(* Logix 5000 AddOnInstructionDefinition export B256_MODINV; software revision 30.00 *)

ADD_ON_INSTRUCTION D_SHR   (* revision 1.0, vendor Ken Fischer, NSWCPD, C512 *)
// DINT bit shift right of the 32-bit argument Inp_A by Inp_B bits with paddding by zeros on the right
// Revision note:
// Rev1.0: TBD - Initial Release
VAR_IN_OUT
   Inp_A : DINT; {required}   // 64-bit Integer to be right circular rotated
END_VAR
VAR_INPUT
   Inp_B : INT; {required}   // Number of bits to shift
END_VAR
VAR_IN_OUT
   Out : DINT; {required}   // Result
END_VAR
VAR
   BSR_Cntrl : CONTROL := (LEN := 32);
   ONS : BOOL;
   Source_Bit : BOOL;
   Wrk_InpA : DINT[2];
END_VAR

ROUTINE Logic   (* ladder *)
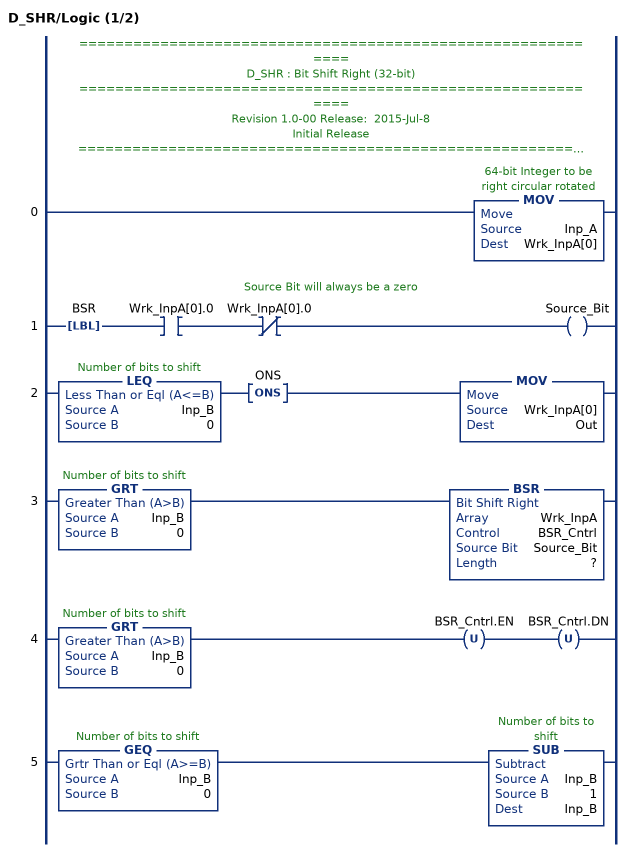
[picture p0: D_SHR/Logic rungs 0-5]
   // ============================================================
   // D_SHR : Bit Shift Right (32-bit)
   // ============================================================
   // Revision 1.0-00 Release:  2015-Jul-8
   // Initial Release
   // ============================================================
   // Performs a right bit shift of the 32-bit argument Inp_A by the
   // number of bits defined in the 16-bit argument Inp_B, with padding by zeros.
   0: MOV(Inp_A,Wrk_InpA[0]);
   // Source Bit will always be a zero
   1: LBL(BSR)XIC(Wrk_InpA[0].0)XIO(Wrk_InpA[0].0)OTE(Source_Bit);
   2: LEQ(Inp_B,0)ONS(ONS)MOV(Wrk_InpA[0],Out);
   3: GRT(Inp_B,0)BSR(Wrk_InpA,BSR_Cntrl,Source_Bit,?);
   4: GRT(Inp_B,0)OTU(BSR_Cntrl.EN)OTU(BSR_Cntrl.DN);
   5: GEQ(Inp_B,0)SUB(Inp_B,1,Inp_B);
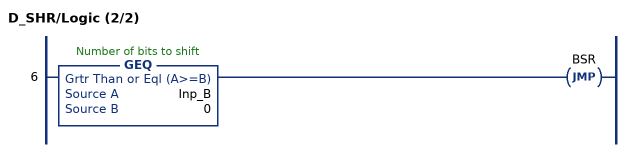
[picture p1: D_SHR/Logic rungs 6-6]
   6: GEQ(Inp_B,0)JMP(BSR);
END_ROUTINE
END_ADD_ON_INSTRUCTION

ADD_ON_INSTRUCTION B256_NRED   (* revision 1.0 20170916, vendor Kenneth A. Fischer *)
// Reduce 256-bit integer stored in 22 pieces by propagating carries
// Revision note:
// Rev1.0: 20170916 - Initial Release
VAR_IN_OUT
   Inp_C : DINT[22]; {required}
END_VAR
VAR
   D_SHR : D_SHR;
   temp : DINT;
   i : INT;
END_VAR

ROUTINE Logic   (* ladder *)
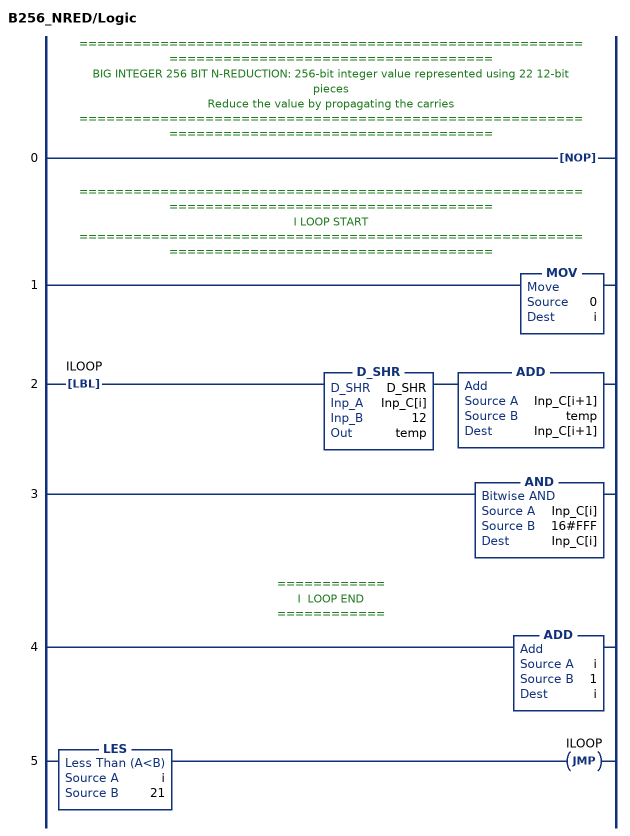
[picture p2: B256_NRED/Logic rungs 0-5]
   // ============================================================================================
   // BIG INTEGER 256 BIT N-REDUCTION: 256-bit integer value represented using 22 12-bit pieces
   // Reduce the value by propagating the carries
   // ============================================================================================
   0: NOP();
   // ============================================================================================
   // I LOOP START
   // ============================================================================================
   1: MOV(0,i);
   2: LBL(ILOOP)D_SHR(D_SHR,Inp_C[i],12,temp)ADD(Inp_C[i+1],temp,Inp_C[i+1]);
   3: AND(Inp_C[i],16#FFF,Inp_C[i]);
   // ============
   // I  LOOP END
   // ============
   4: ADD(i,1,i);
   5: LES(i,21)JMP(ILOOP);
END_ROUTINE
END_ADD_ON_INSTRUCTION

ADD_ON_INSTRUCTION B256_FRED   (* revision 1.0 20170916, vendor Kenneth A. Fischer *)
// fast_reduce:  reduce by propagating the carries starting at a particular offset and stoping once the carry becomes zero
// Revision note:
// Rev1.0: 20170916 - Initial Release
VAR_IN_OUT
   Inp_C : DINT[22]; {required}
END_VAR
VAR_INPUT
   Inp_offset : INT; {required}
END_VAR
VAR
   i : INT;
   carry : DINT;
   D_SHR : D_SHR;
END_VAR

ROUTINE Logic   (* ladder *)
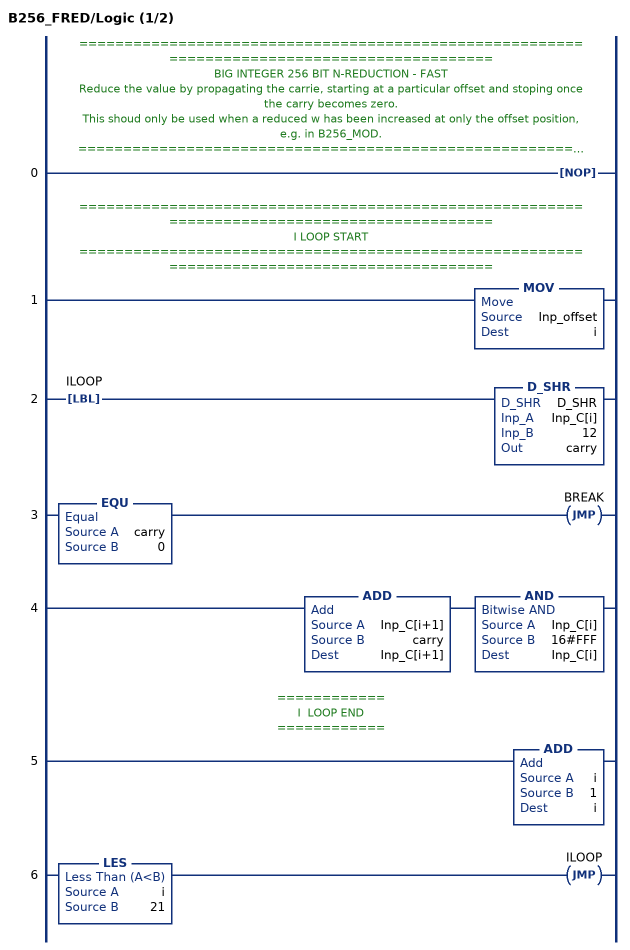
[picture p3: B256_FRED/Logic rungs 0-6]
   // ============================================================================================
   // BIG INTEGER 256 BIT N-REDUCTION - FAST
   // Reduce the value by propagating the carrie, starting at a particular offset and stoping once the carry becomes zero.
   // This shoud only be used when a reduced w has been increased at only the offset position, e.g. in B256_MOD.
   // ============================================================================================
   0: NOP();
   // ============================================================================================
   // I LOOP START
   // ============================================================================================
   1: MOV(Inp_offset,i);
   2: LBL(ILOOP)D_SHR(D_SHR,Inp_C[i],12,carry);
   3: EQU(carry,0)JMP(BREAK);
   4: ADD(Inp_C[i+1],carry,Inp_C[i+1])AND(Inp_C[i],16#FFF,Inp_C[i]);
   // ============
   // I  LOOP END
   // ============
   5: ADD(i,1,i);
   6: LES(i,21)JMP(ILOOP);
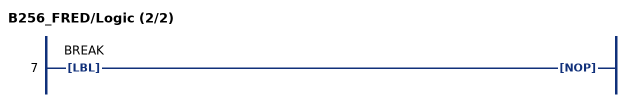
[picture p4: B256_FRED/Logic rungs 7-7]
   7: LBL(BREAK)NOP();
END_ROUTINE
END_ADD_ON_INSTRUCTION

ADD_ON_INSTRUCTION D_SHL   (* revision 1.0, vendor Ken Fischer, NSWCPD, C512 *)
// DINT bit shift left of the 32-bit argument Inp_A by Inp_B bits with paddding by zeros on the right
// Revision note:
// Rev1.0: TBD - Initial Release
VAR_IN_OUT
   Inp_A : DINT; {required}   // 64-bit Integer to be right circular rotated
END_VAR
VAR_INPUT
   Inp_B : INT; {required}   // Number of bits to shift
END_VAR
VAR_IN_OUT
   Out : DINT; {required}   // Result
END_VAR
VAR
   Wrk_InpA : DINT[2];
   Source_Bit : BOOL;
   ONS : BOOL;
   BSL_Cntrl : CONTROL := (LEN := 32);
END_VAR

ROUTINE Logic   (* ladder *)
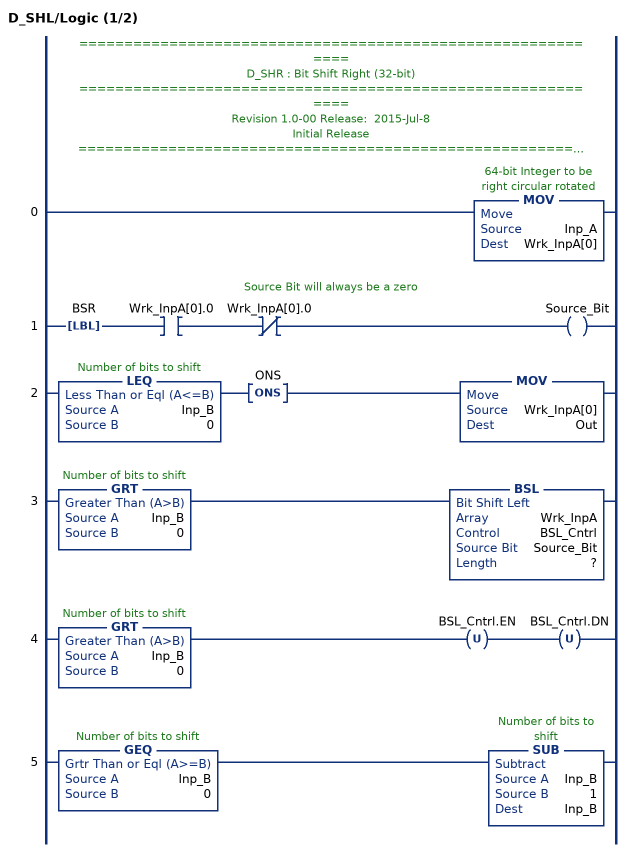
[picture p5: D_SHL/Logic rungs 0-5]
   // ============================================================
   // D_SHR : Bit Shift Right (32-bit)
   // ============================================================
   // Revision 1.0-00 Release:  2015-Jul-8
   // Initial Release
   // ============================================================
   // Performs a left bit shift of the 32-bit argument Inp_A by the
   // number of bits defined in the 16-bit argument Inp_B, with padding by zeros.
   0: MOV(Inp_A,Wrk_InpA[0]);
   // Source Bit will always be a zero
   1: LBL(BSR)XIC(Wrk_InpA[0].0)XIO(Wrk_InpA[0].0)OTE(Source_Bit);
   2: LEQ(Inp_B,0)ONS(ONS)MOV(Wrk_InpA[0],Out);
   3: GRT(Inp_B,0)BSL(Wrk_InpA,BSL_Cntrl,Source_Bit,?);
   4: GRT(Inp_B,0)OTU(BSL_Cntrl.EN)OTU(BSL_Cntrl.DN);
   5: GEQ(Inp_B,0)SUB(Inp_B,1,Inp_B);
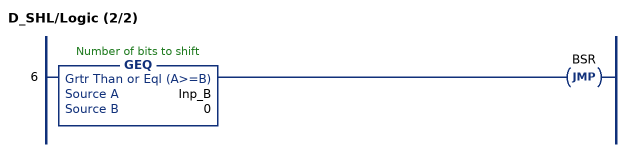
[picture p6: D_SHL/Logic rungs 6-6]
   6: GEQ(Inp_B,0)JMP(BSR);
END_ROUTINE
END_ADD_ON_INSTRUCTION

ADD_ON_INSTRUCTION B256_MOD   (* revision 1.0 20170916, vendor Kenneth A. Fischer *)
// c = d mod (2^255 - 19)
// Revision note:
// Rev1.0: 20170916 - Initial Release
VAR_IN_OUT
   Inp_D : DINT[43]; {required}
   Out_C : DINT[22]; {required}
END_VAR
VAR
   B256_NRED : B256_NRED;
   D_SHL : D_SHL;
   D_SHR : D_SHR;
   i : INT;
   t : DINT;
   temp : DINT;
   temp2 : DINT;
   B256_FRED : B256_FRED;
   offset : DINT;
END_VAR

ROUTINE Logic   (* ladder *)
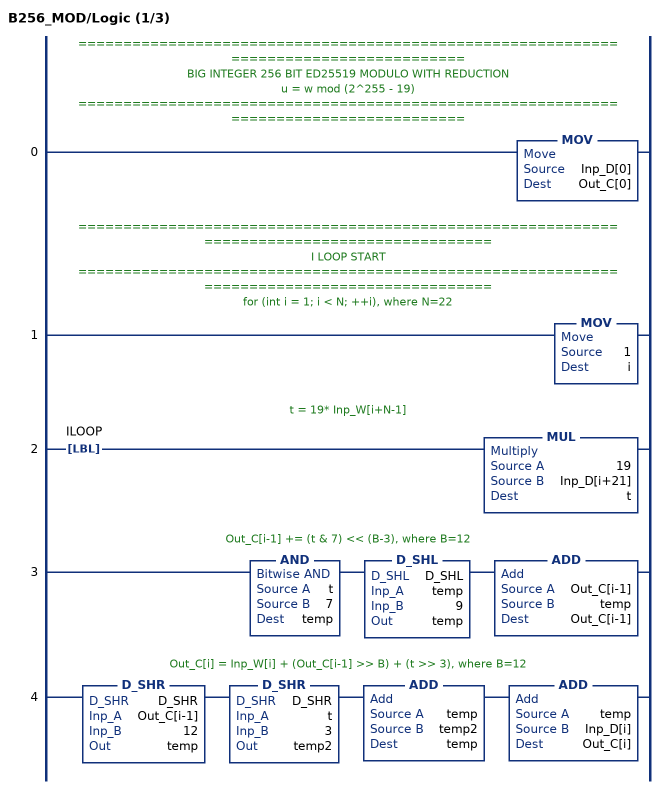
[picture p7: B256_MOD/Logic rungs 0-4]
   // ======================================================================================
   // BIG INTEGER 256 BIT ED25519 MODULO WITH REDUCTION
   //  u = w mod (2^255 - 19)
   // ======================================================================================
   0: MOV(Inp_D[0],Out_C[0]);
   // ============================================================================================
   // I LOOP START
   // ============================================================================================
   // for (int i = 1; i < N; ++i), where N=22
   1: MOV(1,i);
   // t = 19* Inp_W[i+N-1]
   2: LBL(ILOOP)MUL(19,Inp_D[i+21],t);
   // Out_C[i-1] += (t & 7) << (B-3), where B=12
   3: AND(t,7,temp)D_SHL(D_SHL,temp,9,temp)ADD(Out_C[i-1],temp,Out_C[i-1]);
   // Out_C[i] = Inp_W[i] + (Out_C[i-1] >> B) + (t >> 3), where B=12
   4: D_SHR(D_SHR,Out_C[i-1],12,temp)D_SHR(D_SHR,t,3,temp2)ADD(temp,temp2,temp)ADD(temp,Inp_D[i],Out_C[i]);
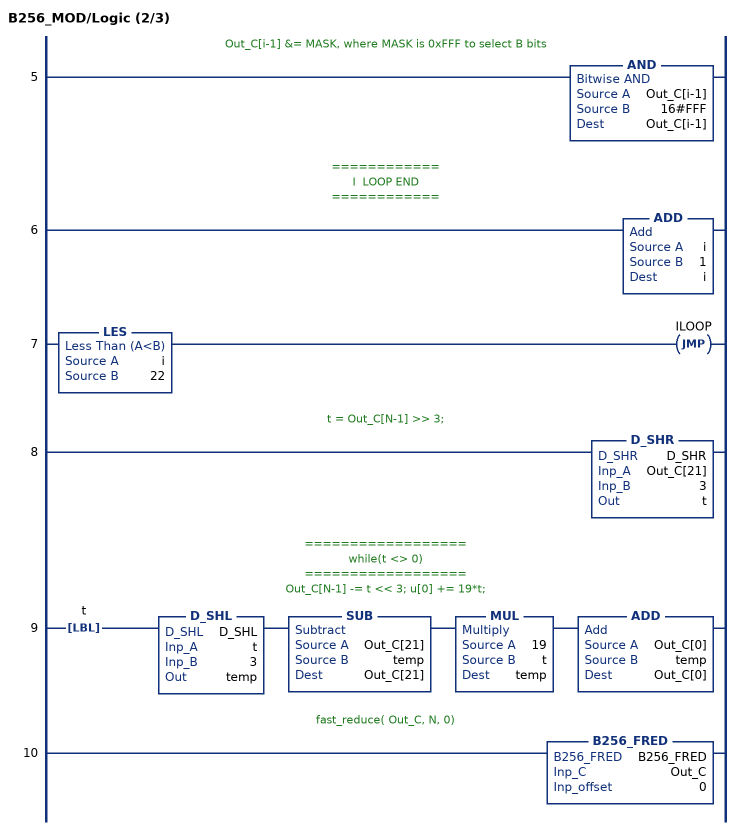
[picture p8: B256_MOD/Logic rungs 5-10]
   // Out_C[i-1] &= MASK, where MASK is 0xFFF to select B bits
   5: AND(Out_C[i-1],16#FFF,Out_C[i-1]);
   // ============
   // I  LOOP END
   // ============
   6: ADD(i,1,i);
   7: LES(i,22)JMP(ILOOP);
   // t = Out_C[N-1] >> 3;
   8: D_SHR(D_SHR,Out_C[21],3,t);
   // ==================
   // while(t <> 0)
   // ==================
   // Out_C[N-1] -= t << 3; u[0] += 19*t;
   9: LBL(t)D_SHL(D_SHL,t,3,temp)SUB(Out_C[21],temp,Out_C[21])MUL(19,t,temp)ADD(Out_C[0],temp,Out_C[0]);
   // fast_reduce( Out_C, N, 0)
   10: B256_FRED(B256_FRED,Out_C,0);
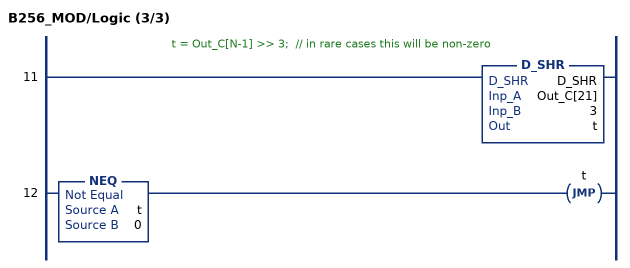
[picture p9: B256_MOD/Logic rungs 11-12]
   // t = Out_C[N-1] >> 3;  // in rare cases this will be non-zero
   11: D_SHR(D_SHR,Out_C[21],3,t);
   12: NEQ(t,0)JMP(t);
END_ROUTINE
END_ADD_ON_INSTRUCTION

ADD_ON_INSTRUCTION B256_NNRED   (* revision 1.0 20170916, vendor Kenneth A. Fischer *)
// Reduce 256-bit integer stored in 43 pieces by propagating carries
// Revision note:
// Rev1.0: 20170916 - Initial Release
VAR_IN_OUT
   Inp_D : DINT[43]; {required}
END_VAR
VAR
   temp : DINT;
   i : INT;
   D_SHR : D_SHR;
END_VAR

ROUTINE Logic   (* ladder *)
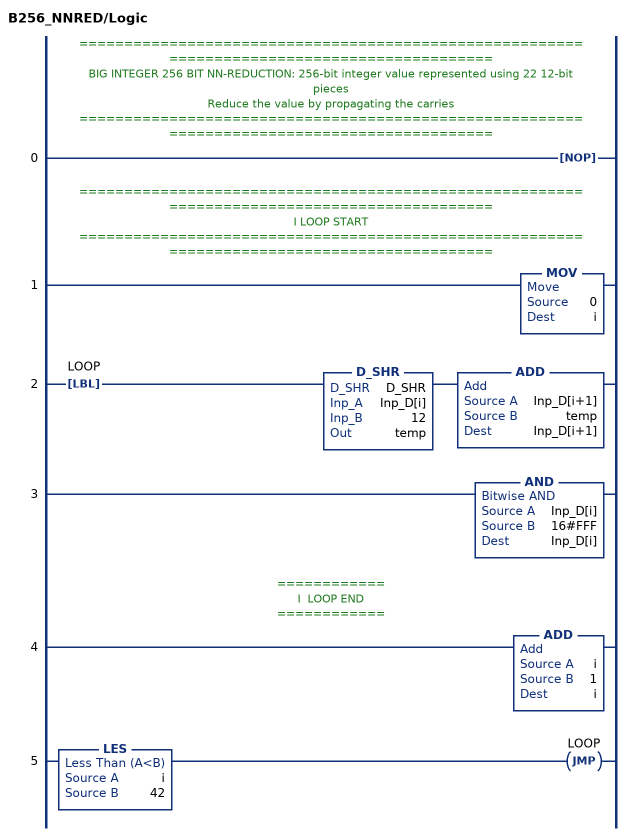
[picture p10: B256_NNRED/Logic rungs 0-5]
   // ============================================================================================
   // BIG INTEGER 256 BIT NN-REDUCTION: 256-bit integer value represented using 22 12-bit pieces
   // Reduce the value by propagating the carries
   // ============================================================================================
   0: NOP();
   // ============================================================================================
   // I LOOP START
   // ============================================================================================
   1: MOV(0,i);
   2: LBL(LOOP)D_SHR(D_SHR,Inp_D[i],12,temp)ADD(Inp_D[i+1],temp,Inp_D[i+1]);
   3: AND(Inp_D[i],16#FFF,Inp_D[i]);
   // ============
   // I  LOOP END
   // ============
   4: ADD(i,1,i);
   5: LES(i,42)JMP(LOOP);
END_ROUTINE
END_ADD_ON_INSTRUCTION

ADD_ON_INSTRUCTION B256_MUL   (* revision 1.0 20170916, vendor Kenneth A. Fischer *)
// c3 = c1*c2 with reduction and mod
// Revision note:
// Rev1.0: 20170916 - Initial Release
VAR_IN_OUT
   Temp_D : DINT[43]; {required}
   Inp_C1 : DINT[22]; {required}
   Inp_C2 : DINT[22]; {required}
   Out_C3 : DINT[22]; {required}
END_VAR
VAR
   B256_MOD : B256_MOD;
   B256_NNRED : B256_NNRED;
   i : INT;
   j : INT;
   mul_temp : DINT;
END_VAR

ROUTINE Logic   (* ladder *)
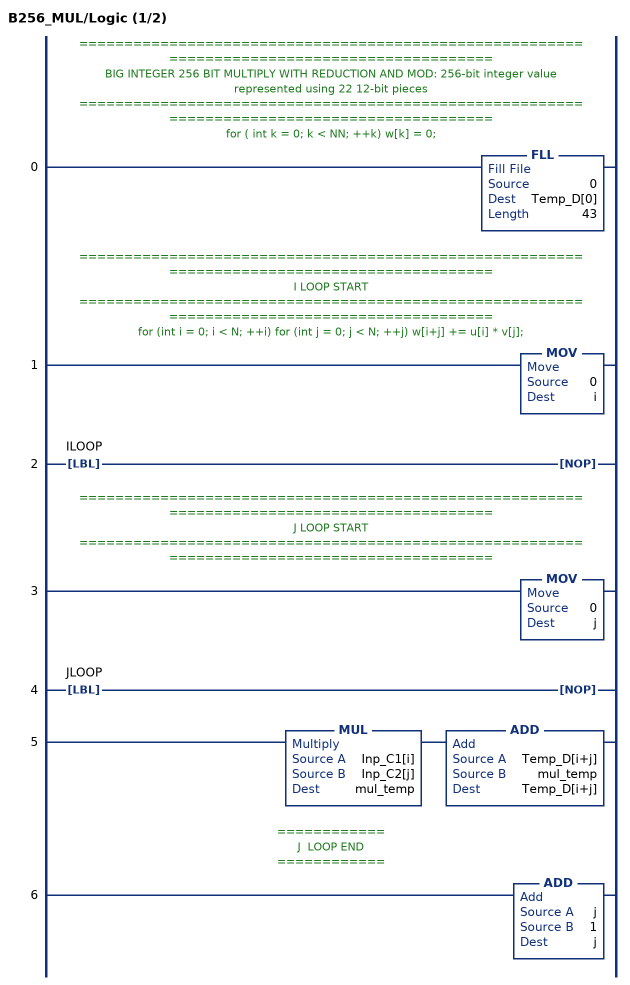
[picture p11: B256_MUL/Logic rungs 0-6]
   // ============================================================================================
   // BIG INTEGER 256 BIT MULTIPLY WITH REDUCTION AND MOD: 256-bit integer value represented using 22 12-bit pieces
   // ============================================================================================
   // for ( int k = 0; k < NN; ++k) w[k] = 0;
   0: FLL(0,Temp_D[0],43);
   // ============================================================================================
   // I LOOP START
   // ============================================================================================
   // for (int i = 0; i < N; ++i) for (int j = 0; j < N; ++j) w[i+j] += u[i] * v[j];
   1: MOV(0,i);
   2: LBL(ILOOP)NOP();
   // ============================================================================================
   // J LOOP START
   // ============================================================================================
   3: MOV(0,j);
   4: LBL(JLOOP)NOP();
   5: MUL(Inp_C1[i],Inp_C2[j],mul_temp)ADD(Temp_D[i+j],mul_temp,Temp_D[i+j]);
   // ============
   // J  LOOP END
   // ============
   6: ADD(j,1,j);
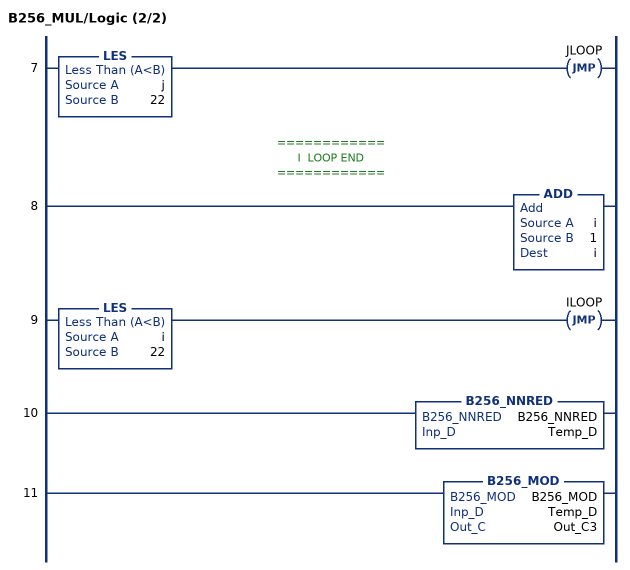
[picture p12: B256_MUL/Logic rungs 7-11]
   7: LES(j,22)JMP(JLOOP);
   // ============
   // I  LOOP END
   // ============
   8: ADD(i,1,i);
   9: LES(i,22)JMP(ILOOP);
   10: B256_NNRED(B256_NNRED,Temp_D);
   11: B256_MOD(B256_MOD,Temp_D,Out_C3);
END_ROUTINE
END_ADD_ON_INSTRUCTION

ADD_ON_INSTRUCTION B256_SQU   (* revision 1.0 20170916, vendor Kenneth A. Fischer *)
// c2 = c1*c1 with reduction and mod
// uses about half the number of multiplies compared to B256_MOD
// Revision note:
// Rev1.0: 20170916 - Initial Release
VAR_IN_OUT
   Temp_D : DINT[43]; {required}
   Inp_C1 : DINT[22]; {required}
   Out_C2 : DINT[22]; {required}
END_VAR
VAR
   B256_NNRED : B256_NNRED;
   i : INT;
   j : INT;
   z : INT;
   mul_temp : DINT;
   B256_MOD : B256_MOD;
   B256_NRED : B256_NRED;
   t : DINT;
END_VAR

ROUTINE Logic   (* ladder *)
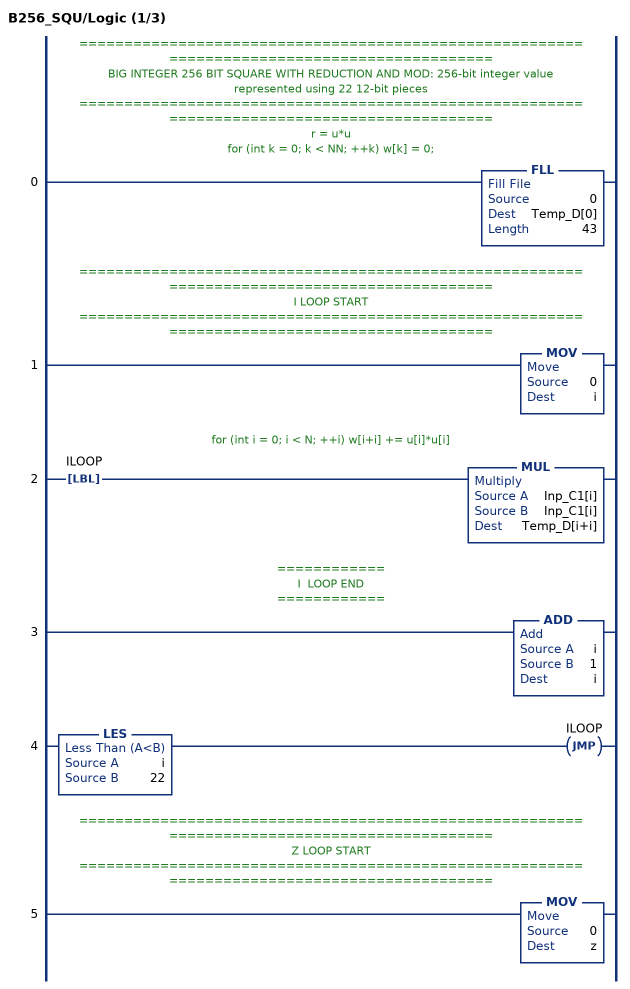
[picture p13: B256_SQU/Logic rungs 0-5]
   // ============================================================================================
   // BIG INTEGER 256 BIT SQUARE WITH REDUCTION AND MOD: 256-bit integer value represented using 22 12-bit pieces
   // ============================================================================================
   // r = u*u
   // for (int k = 0; k < NN; ++k) w[k] = 0;
   0: FLL(0,Temp_D[0],43);
   // ============================================================================================
   // I LOOP START
   // ============================================================================================
   1: MOV(0,i);
   // for (int i = 0; i < N; ++i) w[i+i] += u[i]*u[i]
   2: LBL(ILOOP)MUL(Inp_C1[i],Inp_C1[i],Temp_D[i+i]);
   // ============
   // I  LOOP END
   // ============
   3: ADD(i,1,i);
   4: LES(i,22)JMP(ILOOP);
   // ============================================================================================
   // Z LOOP START
   // ============================================================================================
   5: MOV(0,z);
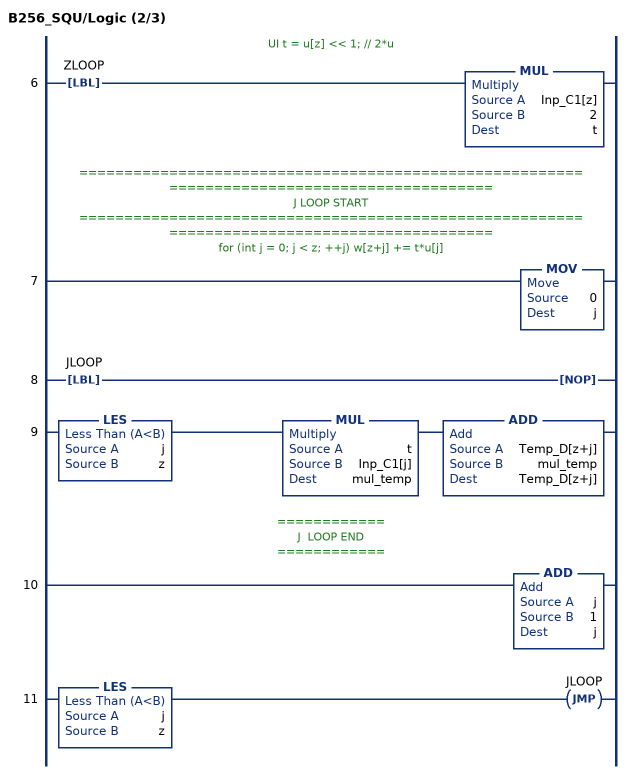
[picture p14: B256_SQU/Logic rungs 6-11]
   // UI t = u[z] << 1; // 2*u
   6: LBL(ZLOOP)MUL(Inp_C1[z],2,t);
   // ============================================================================================
   // J LOOP START
   // ============================================================================================
   // for (int j = 0; j < z; ++j) w[z+j] += t*u[j]
   7: MOV(0,j);
   8: LBL(JLOOP)NOP();
   9: LES(j,z)MUL(t,Inp_C1[j],mul_temp)ADD(Temp_D[z+j],mul_temp,Temp_D[z+j]);
   // ============
   // J  LOOP END
   // ============
   10: ADD(j,1,j);
   11: LES(j,z)JMP(JLOOP);
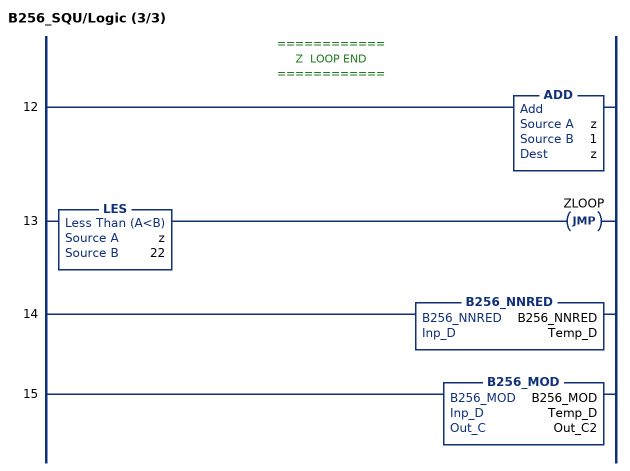
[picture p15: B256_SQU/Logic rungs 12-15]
   // ============
   // Z  LOOP END
   // ============
   12: ADD(z,1,z);
   13: LES(z,22)JMP(ZLOOP);
   14: B256_NNRED(B256_NNRED,Temp_D);
   15: B256_MOD(B256_MOD,Temp_D,Out_C2);
END_ROUTINE
END_ADD_ON_INSTRUCTION

ADD_ON_INSTRUCTION B256_MODINV   (* revision 1.0 20170916, vendor Kenneth A. Fischer *)
// c2 = c1^(m-2) mod m, m=2^255-19
// Revision note:
// Rev1.0: 20170916 - Initial Release
VAR_IN_OUT
   Temp_C1 : DINT[22]; {required}
   Temp_C2 : DINT[22]; {required}
   Temp_D : DINT[43]; {required}
   Temp_E : DINT[32]; {required}
   Inp_C1 : DINT[22]; {required}   // V
   Out_C2 : DINT[22]; {required}   // U
END_VAR
VAR_OUTPUT
   i : INT; {access Read Only}
END_VAR
VAR_INPUT
   SEQCTRL_RESET : BOOL;   // Resets Point Multiplication if Toggled True
END_VAR
VAR_OUTPUT
   SEQCTRL_DN : BOOL; {access Read Only}   // Complete
   SEQCTRL_STEP : INT; {access Read Only}
END_VAR
VAR
   SEQCTRL_CMD : INT;
   SEQCTRL_DONE : INT;
   SEQCTRL_CMD_TABLE : INT[35];
   SEQCTRL_NEXT_STEP : INT;
   TEMP : INT;
   j : INT;
   b : DINT;
   B256_MUL : B256_MUL;
   B256_SQU : B256_SQU;
END_VAR

ROUTINE Logic   (* ladder *)
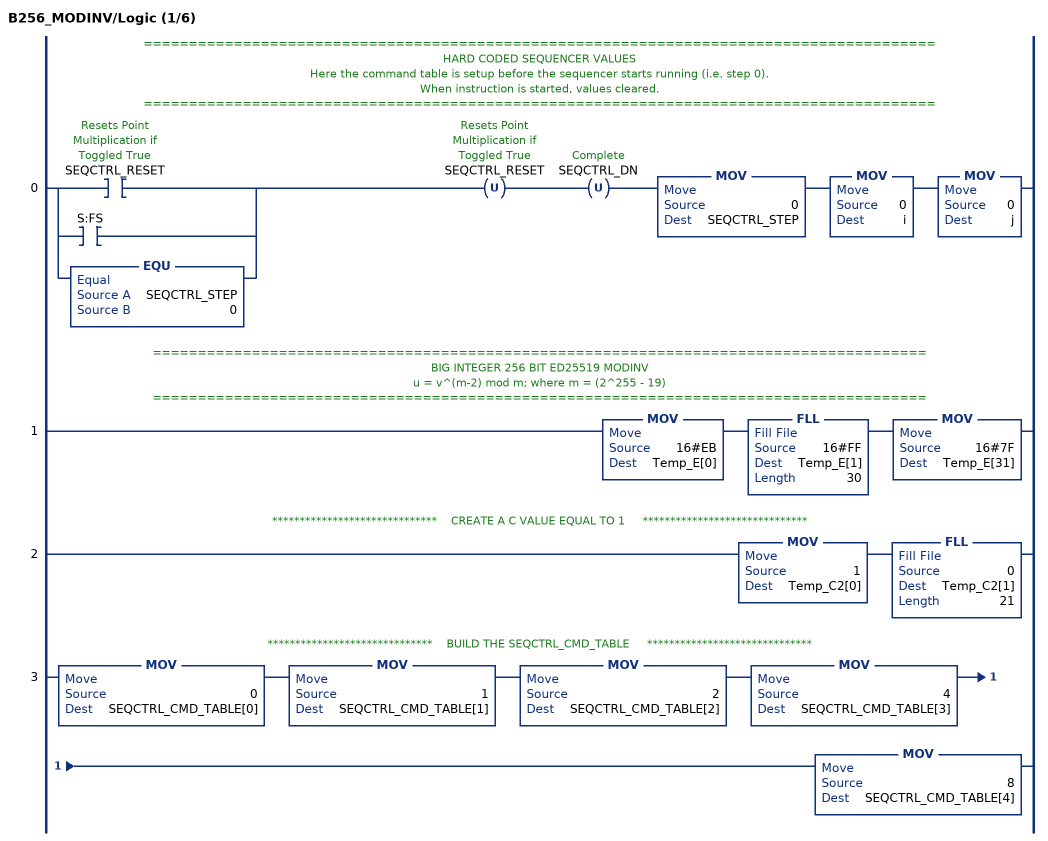
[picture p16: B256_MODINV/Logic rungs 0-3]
   // ========================================================================================
   // HARD CODED SEQUENCER VALUES
   // Here the command table is setup before the sequencer starts running (i.e. step 0).
   // When instruction is started, values cleared.
   // ========================================================================================
   0: [[XIC(SEQCTRL_RESET) ,XIC(S:FS) ] ,EQU(SEQCTRL_STEP,0) ]OTU(SEQCTRL_RESET)OTU(SEQCTRL_DN)MOV(0,SEQCTRL_STEP)MOV(0,i)MOV(0,j);
   // ======================================================================================
   // BIG INTEGER 256 BIT ED25519 MODINV
   //  u = v^(m-2) mod m; where m = (2^255 - 19)
   // ======================================================================================
   1: MOV(16#EB,Temp_E[0])FLL(16#FF,Temp_E[1],30)MOV(16#7F,Temp_E[31]);
   // ******************************    CREATE A C VALUE EQUAL TO 1     ******************************
   2: MOV(1,Temp_C2[0])FLL(0,Temp_C2[1],21);
   // ******************************    BUILD THE SEQCTRL_CMD_TABLE     ******************************
   3: MOV(0,SEQCTRL_CMD_TABLE[0])MOV(1,SEQCTRL_CMD_TABLE[1])MOV(2,SEQCTRL_CMD_TABLE[2])MOV(4,SEQCTRL_CMD_TABLE[3])MOV(8,SEQCTRL_CMD_TABLE[4]);
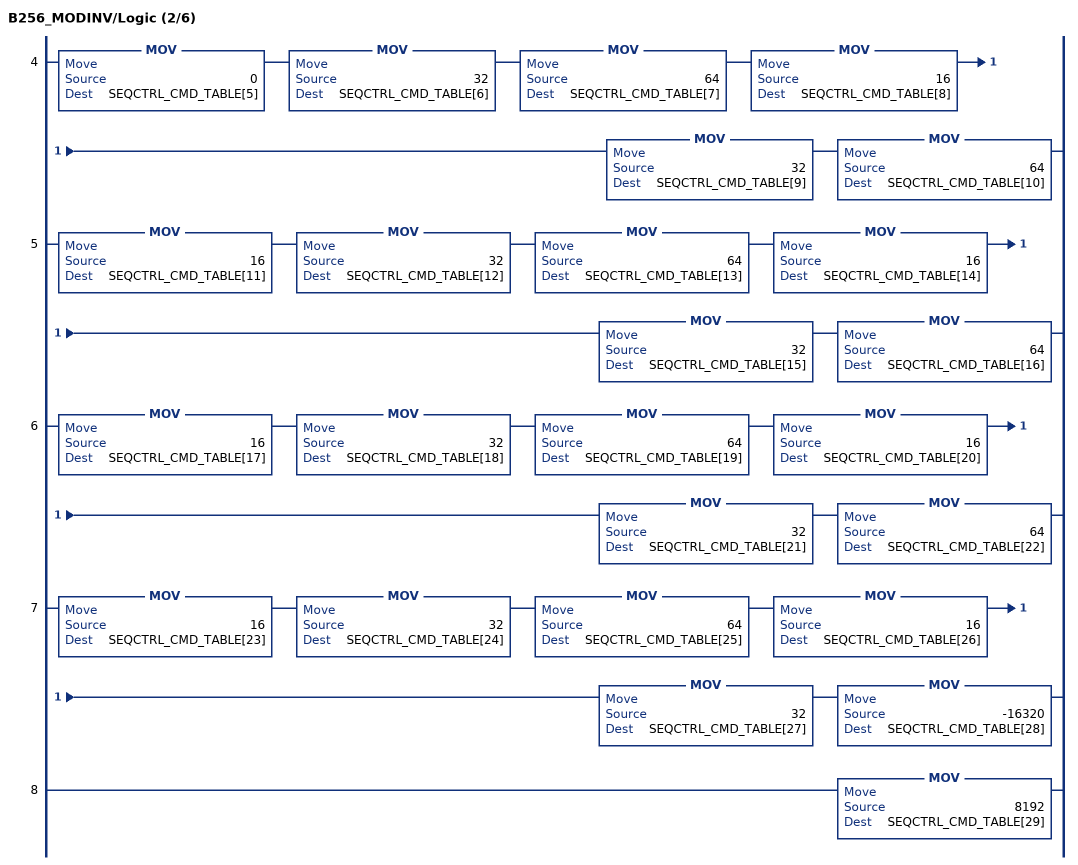
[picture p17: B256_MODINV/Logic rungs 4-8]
   4: MOV(0,SEQCTRL_CMD_TABLE[5])MOV(32,SEQCTRL_CMD_TABLE[6])MOV(64,SEQCTRL_CMD_TABLE[7])MOV(16,SEQCTRL_CMD_TABLE[8])MOV(32,SEQCTRL_CMD_TABLE[9])MOV(64,SEQCTRL_CMD_TABLE[10]);
   5: MOV(16,SEQCTRL_CMD_TABLE[11])MOV(32,SEQCTRL_CMD_TABLE[12])MOV(64,SEQCTRL_CMD_TABLE[13])MOV(16,SEQCTRL_CMD_TABLE[14])MOV(32,SEQCTRL_CMD_TABLE[15])MOV(64,SEQCTRL_CMD_TABLE[16]);
   6: MOV(16,SEQCTRL_CMD_TABLE[17])MOV(32,SEQCTRL_CMD_TABLE[18])MOV(64,SEQCTRL_CMD_TABLE[19])MOV(16,SEQCTRL_CMD_TABLE[20])MOV(32,SEQCTRL_CMD_TABLE[21])MOV(64,SEQCTRL_CMD_TABLE[22]);
   7: MOV(16,SEQCTRL_CMD_TABLE[23])MOV(32,SEQCTRL_CMD_TABLE[24])MOV(64,SEQCTRL_CMD_TABLE[25])MOV(16,SEQCTRL_CMD_TABLE[26])MOV(32,SEQCTRL_CMD_TABLE[27])MOV(-16320,SEQCTRL_CMD_TABLE[28]);
   8: MOV(8192,SEQCTRL_CMD_TABLE[29]);
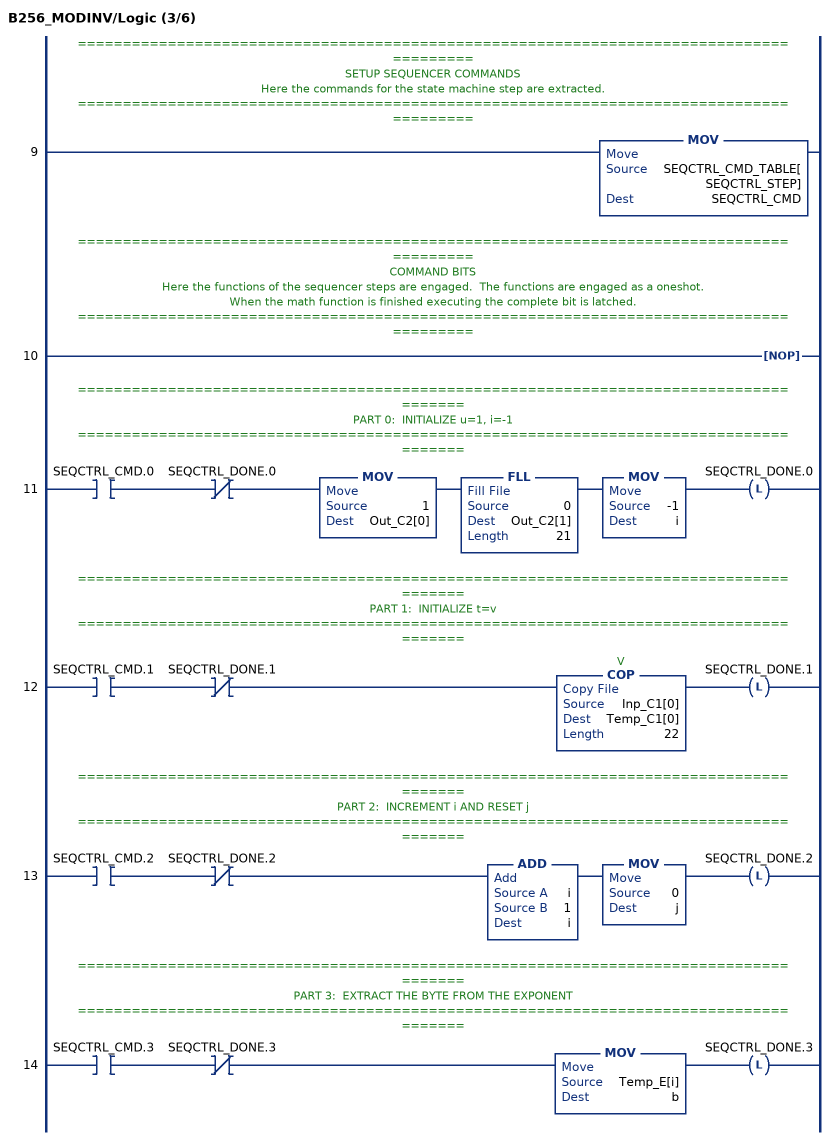
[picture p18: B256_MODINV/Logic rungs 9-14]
   // ========================================================================================
   // SETUP SEQUENCER COMMANDS
   // Here the commands for the state machine step are extracted.
   // ========================================================================================
   9: MOV(SEQCTRL_CMD_TABLE[SEQCTRL_STEP],SEQCTRL_CMD);
   // ========================================================================================
   // COMMAND BITS
   // Here the functions of the sequencer steps are engaged.  The functions are engaged as a oneshot.
   // When the math function is finished executing the complete bit is latched.
   // ========================================================================================
   10: NOP();
   // ======================================================================================
   // PART 0:  INITIALIZE u=1, i=-1
   // ======================================================================================
   11: XIC(SEQCTRL_CMD.0)XIO(SEQCTRL_DONE.0)MOV(1,Out_C2[0])FLL(0,Out_C2[1],21)MOV(-1,i)OTL(SEQCTRL_DONE.0);
   // ======================================================================================
   // PART 1:  INITIALIZE t=v
   // ======================================================================================
   12: XIC(SEQCTRL_CMD.1)XIO(SEQCTRL_DONE.1)COP(Inp_C1[0],Temp_C1[0],22)OTL(SEQCTRL_DONE.1);
   // ======================================================================================
   // PART 2:  INCREMENT i AND RESET j
   // ======================================================================================
   13: XIC(SEQCTRL_CMD.2)XIO(SEQCTRL_DONE.2)ADD(i,1,i)MOV(0,j)OTL(SEQCTRL_DONE.2);
   // ======================================================================================
   // PART 3:  EXTRACT THE BYTE FROM THE EXPONENT
   // ======================================================================================
   14: XIC(SEQCTRL_CMD.3)XIO(SEQCTRL_DONE.3)MOV(Temp_E[i],b)OTL(SEQCTRL_DONE.3);
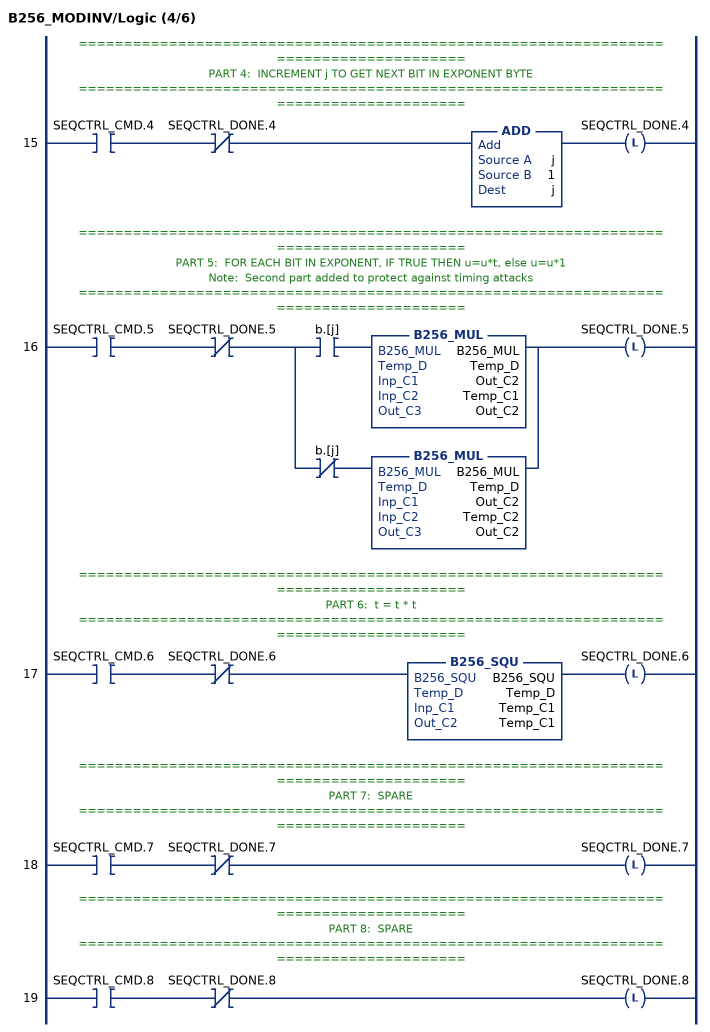
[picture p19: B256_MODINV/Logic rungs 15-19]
   // ======================================================================================
   // PART 4:  INCREMENT j TO GET NEXT BIT IN EXPONENT BYTE
   // ======================================================================================
   15: XIC(SEQCTRL_CMD.4)XIO(SEQCTRL_DONE.4)ADD(j,1,j)OTL(SEQCTRL_DONE.4);
   // ======================================================================================
   // PART 5:  FOR EACH BIT IN EXPONENT, IF TRUE THEN u=u*t, else u=u*1
   // Note:  Second part added to protect against timing attacks
   // ======================================================================================
   16: XIC(SEQCTRL_CMD.5)XIO(SEQCTRL_DONE.5)[XIC(b.[j]) B256_MUL(B256_MUL,Temp_D,Out_C2,Temp_C1,Out_C2) ,XIO(b.[j]) B256_MUL(B256_MUL,Temp_D,Out_C2,Temp_C2,Out_C2) ]OTL(SEQCTRL_DONE.5);
   // ======================================================================================
   // PART 6:  t = t * t
   // ======================================================================================
   17: XIC(SEQCTRL_CMD.6)XIO(SEQCTRL_DONE.6)B256_SQU(B256_SQU,Temp_D,Temp_C1,Temp_C1)OTL(SEQCTRL_DONE.6);
   // ======================================================================================
   // PART 7:  SPARE
   // ======================================================================================
   18: XIC(SEQCTRL_CMD.7)XIO(SEQCTRL_DONE.7)OTL(SEQCTRL_DONE.7);
   // ======================================================================================
   // PART 8:  SPARE
   // ======================================================================================
   19: XIC(SEQCTRL_CMD.8)XIO(SEQCTRL_DONE.8)OTL(SEQCTRL_DONE.8);
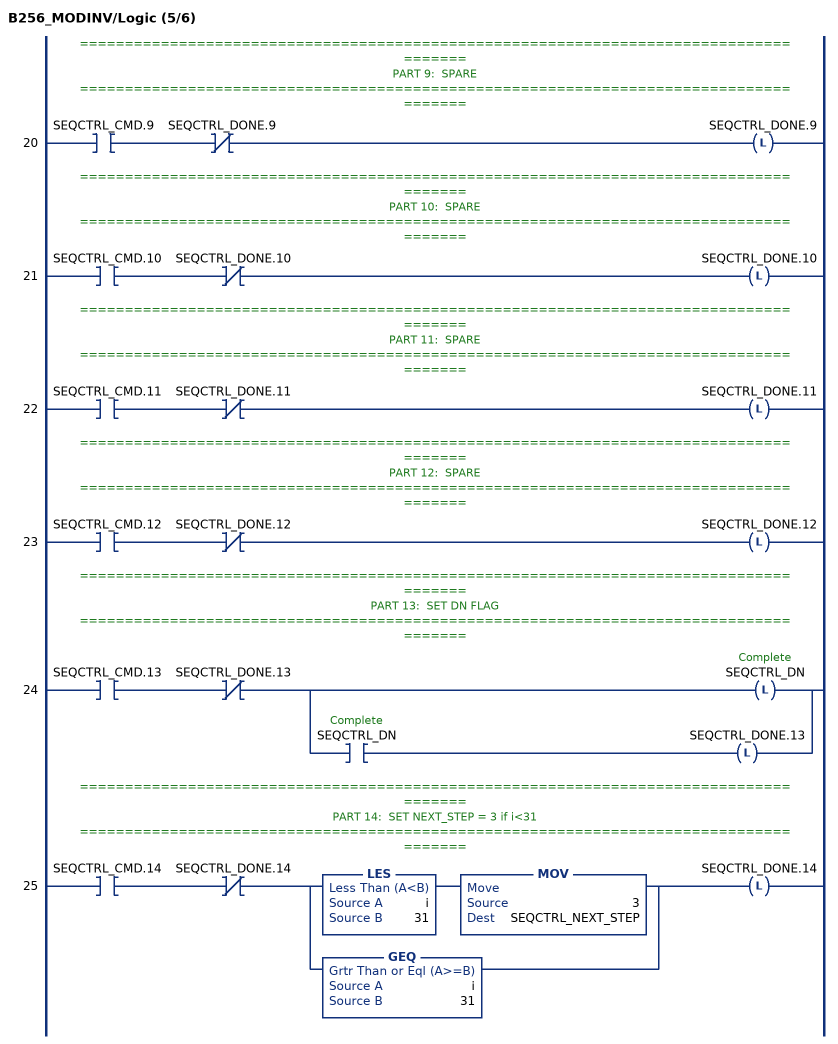
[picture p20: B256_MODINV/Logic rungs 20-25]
   // ======================================================================================
   // PART 9:  SPARE
   // ======================================================================================
   20: XIC(SEQCTRL_CMD.9)XIO(SEQCTRL_DONE.9)OTL(SEQCTRL_DONE.9);
   // ======================================================================================
   // PART 10:  SPARE
   // ======================================================================================
   21: XIC(SEQCTRL_CMD.10)XIO(SEQCTRL_DONE.10)OTL(SEQCTRL_DONE.10);
   // ======================================================================================
   // PART 11:  SPARE
   // ======================================================================================
   22: XIC(SEQCTRL_CMD.11)XIO(SEQCTRL_DONE.11)OTL(SEQCTRL_DONE.11);
   // ======================================================================================
   // PART 12:  SPARE
   // ======================================================================================
   23: XIC(SEQCTRL_CMD.12)XIO(SEQCTRL_DONE.12)OTL(SEQCTRL_DONE.12);
   // ======================================================================================
   // PART 13:  SET DN FLAG
   // ======================================================================================
   24: XIC(SEQCTRL_CMD.13)XIO(SEQCTRL_DONE.13)[OTL(SEQCTRL_DN) ,XIC(SEQCTRL_DN) OTL(SEQCTRL_DONE.13) ];
   // ======================================================================================
   // PART 14:  SET NEXT_STEP = 3 if i<31
   // ======================================================================================
   25: XIC(SEQCTRL_CMD.14)XIO(SEQCTRL_DONE.14)[LES(i,31) MOV(3,SEQCTRL_NEXT_STEP) ,GEQ(i,31) ]OTL(SEQCTRL_DONE.14);
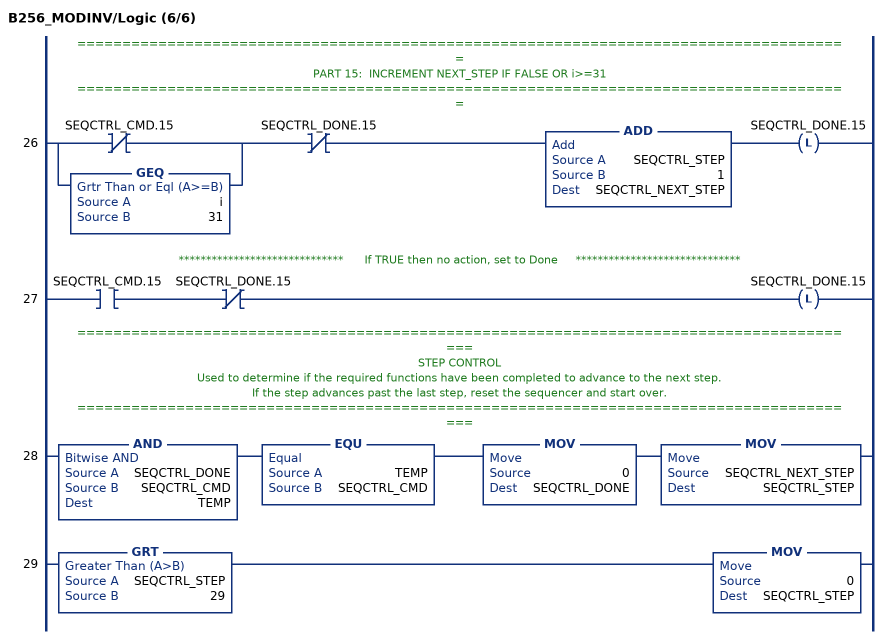
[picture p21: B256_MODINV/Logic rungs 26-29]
   // ======================================================================================
   // PART 15:  INCREMENT NEXT_STEP IF FALSE OR i>=31
   // ======================================================================================
   26: [XIO(SEQCTRL_CMD.15) ,GEQ(i,31) ]XIO(SEQCTRL_DONE.15)ADD(SEQCTRL_STEP,1,SEQCTRL_NEXT_STEP)OTL(SEQCTRL_DONE.15);
   // ******************************      If TRUE then no action, set to Done     ******************************
   27: XIC(SEQCTRL_CMD.15)XIO(SEQCTRL_DONE.15)OTL(SEQCTRL_DONE.15);
   // ========================================================================================
   // STEP CONTROL
   // Used to determine if the required functions have been completed to advance to the next step.
   // If the step advances past the last step, reset the sequencer and start over.
   // ========================================================================================
   28: AND(SEQCTRL_DONE,SEQCTRL_CMD,TEMP)EQU(TEMP,SEQCTRL_CMD)MOV(0,SEQCTRL_DONE)MOV(SEQCTRL_NEXT_STEP,SEQCTRL_STEP);
   29: GRT(SEQCTRL_STEP,29)MOV(0,SEQCTRL_STEP);
END_ROUTINE
END_ADD_ON_INSTRUCTION
